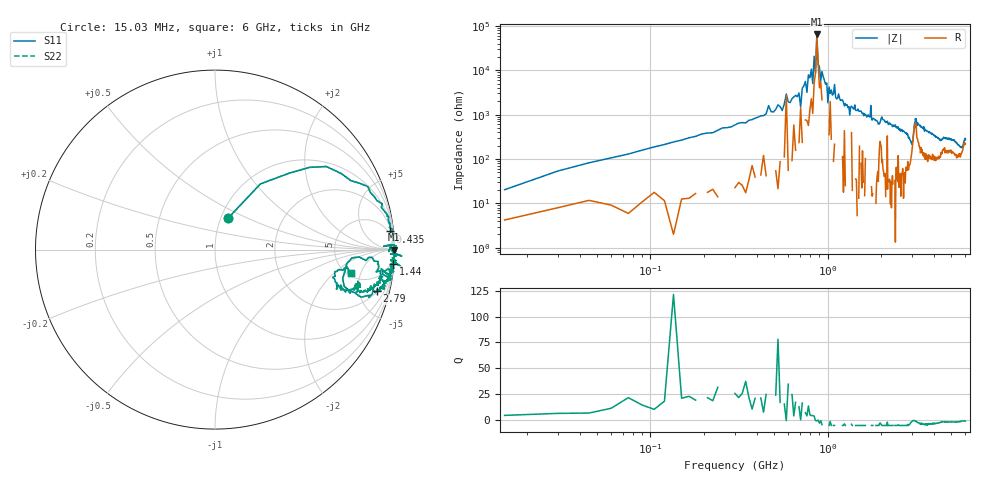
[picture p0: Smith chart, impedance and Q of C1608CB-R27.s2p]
!	Network	Analyzer	HP8753E.07.74:	Oct	30	2002	Serial	No.	JP38451487
!	Hewlett-Packard
!	28	Aug	2009	8:35:38
!	Frequency	S11	S21	S12	S22
#	HZ	S	RI	R	50
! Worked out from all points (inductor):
!   400 points, 15.03 MHz to 6 GHz, reference 50 ohm
!   read as one part in series: L = 276 nH near 45.03 MHz
!   highest |Z| = 64.2 kohm at 870 MHz (marker M1)
!   self-resonance near 570 MHz
!   S11 on the Smith chart (normalised r, x): 15.03 MHz: 1.08, +0.40; 435 MHz: 3, +19; 1.44 GHz: 2, -25; 2.79 GHz: 2.11, -7.29; 6 GHz: 5.40, -3.52
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1.502992e7  0.0737 0.176  0.926 -0.176  0.926 -0.176  0.0737 0.176
1.350293e8  0.852 0.351  0.148 -0.351  0.148 -0.351  0.852 0.351
4.350278e8  0.976 0.101  0.0237 -0.101  0.0237 -0.101  0.976 0.101
5.850271e8  0.968 -0.0103  0.0316 0.0103  0.0316 0.0103  0.968 -0.0103
7.050265e8  0.94 0.0186  0.0605 -0.0186  0.0605 -0.0186  0.94 0.0186
8.10026e8  0.998 0.00916  0.00211 -0.00916  0.00211 -0.00916  0.998 0.00916
8.250259e8  0.995 0.0193  0.00458 -0.0193  0.00458 -0.0193  0.995 0.0193
8.400258e8  0.999 0.00467  0.00122 -0.00467  0.00122 -0.00467  0.999 0.00467
8.550257e8  0.989 -0.00284  0.0107 0.00284  0.0107 0.00284  0.989 -0.00284
8.700256e8  0.999 -0.000885  0.00128 0.000885  0.00128 0.000885  0.999 -0.000885
9.150254e8  0.984 -0.00528  0.0159 0.00528  0.0159 0.00528  0.984 -0.00528
9.90025e8  1 -0.0194  -0.00054 0.0194  -0.00054 0.0194  1 -0.0194
1.005025e9  1.04 -0.0356  -0.0438 0.0356  -0.0438 0.0356  1.04 -0.0356
1.020025e9  0.997 -0.0236  0.00256 0.0236  0.00256 0.0236  0.997 -0.0236
1.440023e9  0.991 -0.079  0.00855 0.079  0.00855 0.079  0.991 -0.079
2.01002e9  0.961 -0.109  0.0394 0.109  0.0394 0.109  0.961 -0.109
2.790016e9  0.901 -0.232  0.099 0.232  0.099 0.232  0.901 -0.232
3.015015e9  0.724 -0.121  0.276 0.121  0.276 0.121  0.724 -0.121
3.135014e9  0.91 -0.0663  0.0903 0.0663  0.0903 0.0663  0.91 -0.0663
4.00501e9  0.864 -0.228  0.136 0.228  0.136 0.228  0.864 -0.228
5.010005e9  0.788 -0.202  0.212 0.202  0.212 0.202  0.788 -0.202
6e9  0.76 -0.132  0.24 0.132  0.24 0.132  0.76 -0.132
